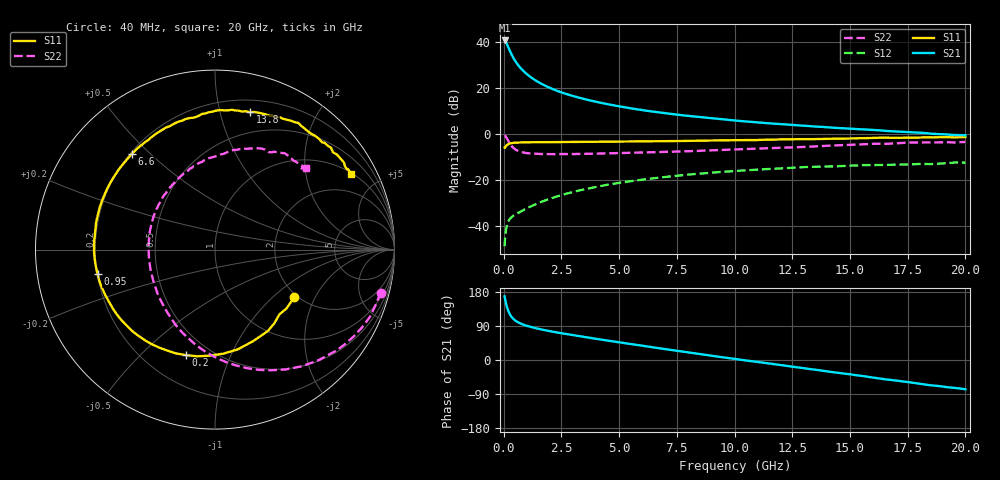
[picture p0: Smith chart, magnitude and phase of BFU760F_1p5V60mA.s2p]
! Filename:  P:\Prog\Test\Noise\ATS_data\Testdata_Net\Split files Spar\BFU760F_2W_C1_Bias8_1.5V_5mA_60mA_D.s2p
! Date/Time: Mon 06/Feb/2012 15:07:47
! BFU760_2W_C1_Bias8_1.5V_5mA_60mA_R.s2p
! MDIF S-parameter v. bias file
! BFU760_2W_C1_1.5V_5mA_60mA
! Date/time Fri Mar 18 11:09:37 2011
! VAR V_out= 1.5000
! VAR I_out= 60.0150
! VAR V_in= 0.8101
! VAR I_in= 0.2191
! Device data file deembeded for feedlines and parallel
! Original file: \Split files Spar\BFU760_2W_C1_Bias8_1.5V_5mA_60mA_R.s2p
! Feed-files: PR003V01_101208_Feed1.s2p, PR003V01_101208_Feed2.s2p
! Parallel-file: PR003V01_101208_Par.s2p
# MHz S MA R 50
!  Freq-MHz  S11-mag  S11-arg  S21-mag  S21-arg  S12-mag  S12-arg  S22-mag  S22-arg
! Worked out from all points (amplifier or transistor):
!   167 points, 40 MHz to 20 GHz, reference 50 ohm
!   highest |S21| = 40.7 dB at 40 MHz (marker M1)
!   |S21| within 3 dB of that: start of sweep to 200.5 MHz
!   unconditionally stable (mu >= 1): 2.804 GHz to 15.01 GHz
!   at 550 MHz: K = 0.53, MSG = 32.8 dB, |S12| = -34.6 dB
!   at 4.2 GHz: K = 1.03, MAG = 17.0 dB, |S12| = -22.5 dB
!   at 20 GHz: K = 0.95, MSG = 5.9 dB, |S12| = -12.3 dB
!   S11 on the Smith chart (normalised r, x): 40 MHz: 1.93, -1.39; 200 MHz: 0.37, -0.69; 950 MHz: 0.20, -0.10; 6.6 GHz: 0.21, +0.44; 13.8 GHz: 0.30, +1.24; 20 GHz: 1.04, +3.58
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40  0.5148 -30.8  108.9 167.9  0.003719 80.6  0.9544 -14.6
50  0.5162 -39.5  107 163.8  0.004857 82.3  0.946 -19.5
60  0.509 -45.1  102.8 161.0  0.005552 75.7  0.9405 -23.6
80  0.541 -57.0  103.5 155.0  0.006879 71.1  0.912 -32.0
120  0.5705 -77.3  95.52 144.5  0.0094 63.5  0.8441 -46.9
160  0.5918 -93.0  86.01 136.1  0.01132 57.6  0.7746 -59.5
200  0.6099 -105.4  77.2 129.3  0.01278 53.4  0.7111 -70.3
240  0.6221 -115.4  69.33 123.8  0.0139 50.4  0.6565 -79.6
300  0.6379 -126.9  59.38 117.2  0.01519 47.4  0.5922 -91.3
440  0.6537 -143.9  43.69 107.2  0.01733 45.0  0.497 -111.5
650  0.6614 -157.6  30.69 98.6  0.02003 46.1  0.4296 -130.7
950  0.6684 -168.3  21.32 91.2  0.024 49.4  0.3932 -147.4
1300  0.6727 -176.2  15.67 85.2  0.029 52.2  0.3784 -159.6
1800  0.6748 175.9  11.33 78.5  0.03666 54.2  0.3713 -171.0
3400  0.6842 158.7  5.979 61.8  0.06232 51.7  0.3752 167.0
6600  0.7066 130.8  3.042 32.3  0.1126 34.9  0.4088 136.6
6800  0.7079 129.2  2.953 30.5  0.1155 33.5  0.4116 134.8
10200  0.7457 102.6  1.951 1.3  0.1615 11.3  0.472 107.3
13400  0.7836 78.9  1.482 -24.9  0.1969 -11.0  0.5422 83.7
13800  0.79 75.8  1.447 -28.2  0.1998 -13.9  0.5552 81.0
16800  0.8391 53.4  1.162 -52.8  0.2179 -33.3  0.628 59.7
20000  0.8685 29.1  0.9491 -77.3  0.2427 -54.9  0.6809 41.7
